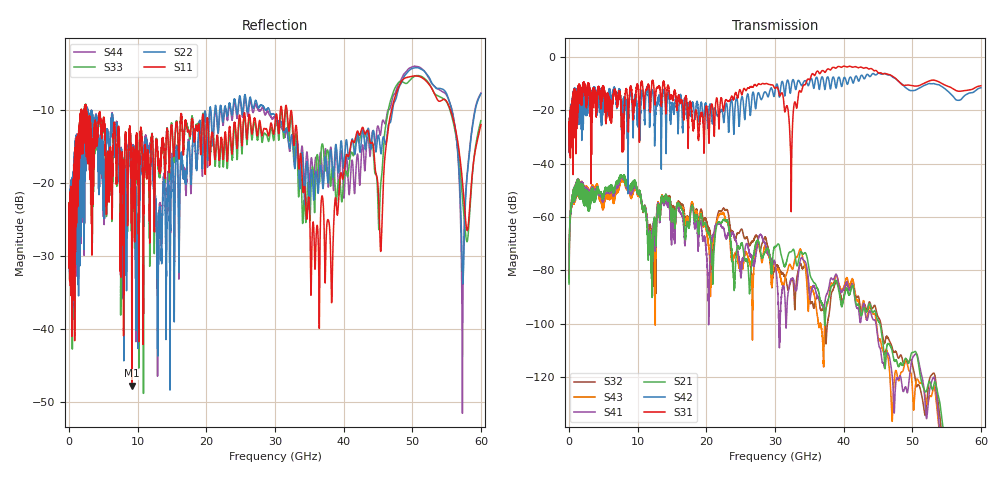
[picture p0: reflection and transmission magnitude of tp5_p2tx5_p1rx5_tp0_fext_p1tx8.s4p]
! 100G CR Analysis
! File: tp5_p2tx5_p1rx5_tp0_fext_p2tx8
! Description: 2m Cu Cable, OSFP, TP0-TP5
! Port Mapping
! Port1 -- P1RX5N
! Port2 -- P2TX8N
! Port3 -- P1RX5P
! Port4 -- P2TX8P
# GHz S MA R 50.00
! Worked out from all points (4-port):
!   6000 points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, 10 MHz to 60 GHz, reference 50 ohm
!   strongest paths, dB at 10 MHz, 15.01 GHz, 30.01 GHz, 45.01 GHz, 60 GHz:
!     S31: -28.1, -15.5, -11.8, -5.9, -10.8
!     S42: -27.9, -18.4, -12.9, -6.2, -11.6
!     S21: -85.1, -58.2, -71.0, -98.8, -176.4
!     S41: -77.2, -61.3, -77.4, -105.8, -172.6
!     S43: -82.7, -59.6, -77.4, -105.6, -173.5
!     S32: -84.5, -57.3, -79.1, -97.4, -192.8
!   lowest |S11| = -47.8 dB at 9.18 GHz (marker M1), VSWR 1.01, Z = 50.3 - j0.299 ohm
!   |S11| at or under -10 dB: 2.505 GHz to 30.79 GHz (28.28 GHz wide, 170 % of centre); 31.75 GHz to 46.99 GHz (15.23 GHz wide, 38.7 % of centre); 55.58 GHz to end of sweep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
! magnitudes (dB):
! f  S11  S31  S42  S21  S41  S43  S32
! 10 MHz  -23.8  -28.1  -27.9  -85.1  -77.2  -82.7  -84.5
! 9.18 GHz  -47.8  -14.2  -17.5  -49.6  -50.8  -52.1  -50.4
! 11.82 GHz  -21.0  -19.4  -20.3  -66.4  -67.2  -65.7  -63.1
! 38.25 GHz  -36.4  -4.4  -9.6  -85.7  -82.9  -84.7  -88.4
! 50.9 GHz  -5.3  -10.8  -11.9  -114.8  -113.5  -121.3  -122.7
! 57.32 GHz  -19.9  -12.8  -15.4  -169.0  -172.6  -160.4  -167.6
! 60 GHz  -12.0  -10.8  -11.6  -176.4  -172.6  -173.5  -192.8
